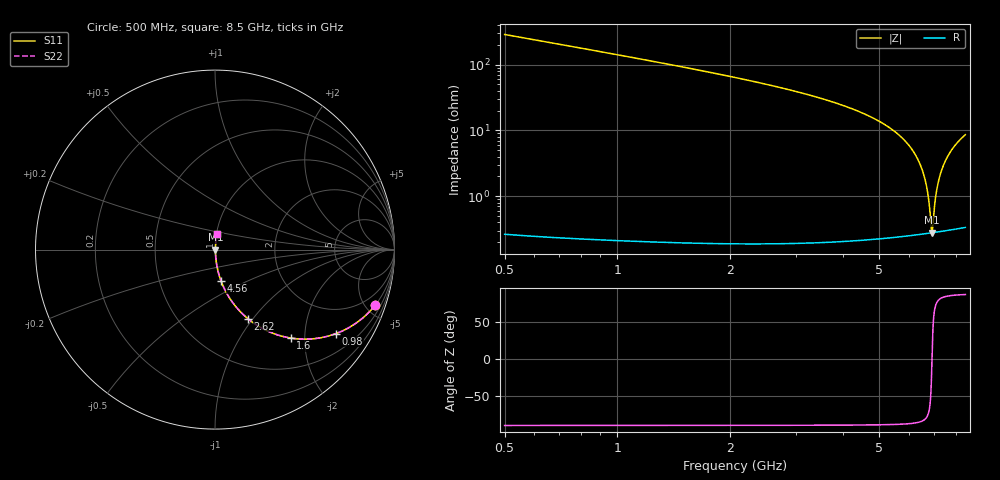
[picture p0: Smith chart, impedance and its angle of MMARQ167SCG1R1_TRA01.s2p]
! MMARQ167SCG1R1_TRA01  S-PARAMETER MODEL  ( General Type )
! Model Generated by TAIYO YUDEN Corporation (http://www.ty-top.com)
! Version 1.0
! TAIYO YUDEN Control No. 160201
! Copyright(c) 2016 TAIYO YUDEN CO.,LTD. All Rights Reserved.
! Product Description (link to TY-COMPAS)
! https://ds.yuden.co.jp/TYCOMPAS/or/detail?pn=MMARQ167SCG1R1BTRA01&u=M
! Products Name : Multilayer Ceramic Capacitors
! Characteristics :
!  Capacitance : 1.1 pF , Rated Voltage : 250V , TCC : CG / C0G
!  Case Size : 1.6 x 0.8 / 0.063 x 0.031 [mm/inch] , Thickness : 0.7 / 0.028 [mm/inch]
!  (Conditions: Temperature = 25 degC , DC Bias Current/Voltage = 0A / 0V)
! External Node Assignments :
!  1  o---| |---o  2
! GND o---------o GND
! Frequency Range : 500MHz  -  8500MHz  [ 401 STEP ]
# MHz S RI R 50
! Freq[MHz].  S11 Real  S11 Imag  S21 Real  S21 Imag  S12 Real  S12 Imag  S22 Real  S22 Imag
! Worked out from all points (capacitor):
!   401 points, 500 MHz to 8.5 GHz, reference 50 ohm
!   read as one part in series: C = 1.1 pF near 540 MHz
!   lowest |Z| = 278 mohm at 6.92 GHz (marker M1)
!   series resonance near 6.922 GHz, so ESL is about 480 pH
!   S11 on the Smith chart (normalised r, x): 500 MHz: 1.01, -5.74; 980 MHz: 1.00, -2.88; 1.6 GHz: 1.00, -1.71; 2.62 GHz: 1.00, -0.94; 4.56 GHz: 1.00, -0.36; 8.5 GHz: 1.01, +0.17
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500  0.8914 -0.3107  0.1086 0.3107  0.1086 0.3107  0.8914 -0.3107
980  0.6749 -0.4677  0.3251 0.4677  0.3251 0.4677  0.6749 -0.4677
1600  0.4213 -0.4926  0.5787 0.4926  0.5787 0.4926  0.4213 -0.4926
1840  0.3469 -0.4747  0.6531 0.4747  0.6531 0.4747  0.3469 -0.4747
2620  0.1828 -0.3845  0.8172 0.3845  0.8172 0.3845  0.1828 -0.3845
3180  0.1147 -0.316  0.8853 0.316  0.8853 0.316  0.1147 -0.316
4500  0.035 -0.1781  0.965 0.1781  0.965 0.1781  0.035 -0.1781
4560  0.033 -0.1727  0.967 0.1727  0.967 0.1727  0.033 -0.1727
5840  0.00745 -0.0704  0.9926 0.0704  0.9926 0.0704  0.00745 -0.0704
6260  0.00431 -0.0416  0.9957 0.0416  0.9957 0.0416  0.00431 -0.0416
6560  0.00316 -0.0222  0.9968 0.0222  0.9968 0.0222  0.00316 -0.0222
6740  0.00284 -0.011  0.9972 0.011  0.9972 0.011  0.00284 -0.011
6800  0.00279 -0.00734  0.9972 0.00734  0.9972 0.00734  0.00279 -0.00734
6880  0.00277 -0.0025  0.9972 0.0025  0.9972 0.0025  0.00277 -0.0025
6920  0.00278 -9.97e-05  0.9972 9.97e-05  0.9972 9.97e-05  0.00278 -9.97e-05
6960  0.00279 0.00229  0.9972 -0.00229  0.9972 -0.00229  0.00279 0.00229
7080  0.00292 0.00936  0.9971 -0.00936  0.9971 -0.00936  0.00292 0.00936
7180  0.00309 0.0152  0.9969 -0.0152  0.9969 -0.0152  0.00309 0.0152
7380  0.00364 0.0265  0.9964 -0.0265  0.9964 -0.0265  0.00364 0.0265
7660  0.0048 0.0419  0.9952 -0.0419  0.9952 -0.0419  0.0048 0.0419
8040  0.00703 0.0619  0.993 -0.0619  0.993 -0.0619  0.00703 0.0619
8500  0.0106 0.0849  0.9894 -0.0849  0.9894 -0.0849  0.0106 0.0849
